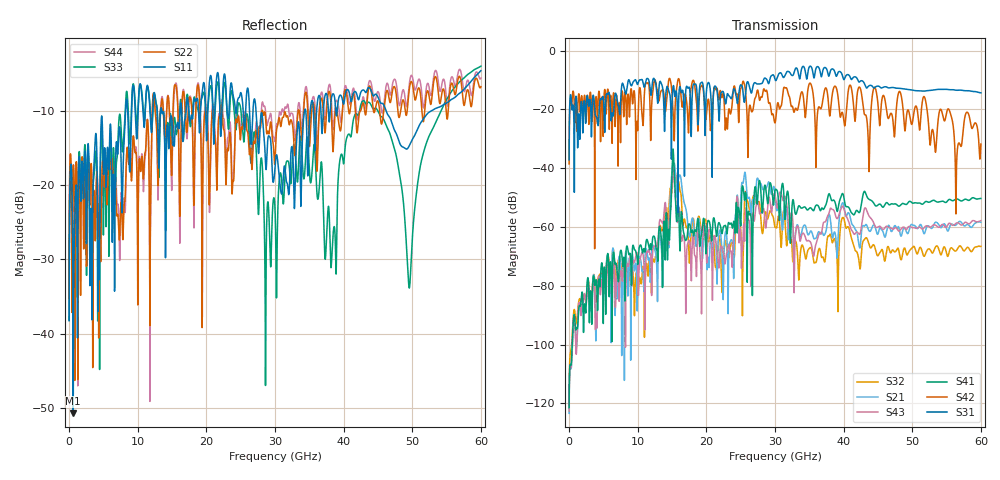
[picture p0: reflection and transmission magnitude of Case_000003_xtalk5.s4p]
! Info: Touchstone file created by circ.  Input file=CasetestDOE_NRZ_template_000003.circ
# Hz S RI R 50
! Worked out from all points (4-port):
!   6000 points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, 10 MHz to 60 GHz, reference 50 ohm
!   strongest paths, dB at 10 MHz, 15.01 GHz, 30.01 GHz, 45.01 GHz, 60 GHz:
!     S31: -37.1, -18.3, -9.8, -12.1, -14.4
!     S42: -38.6, -14.8, -24.6, -18.3, -31.8
!     S41: -121.4, -40.7, -47.5, -52.5, -50.3
!     S43: -122.6, -43.5, -49.2, -60.0, -57.9
!     S21: -123.4, -40.4, -48.7, -62.3, -58.4
!     S32: -120.6, -46.8, -60.1, -69.8, -66.6
!   lowest |S11| = -50.7 dB at 610 MHz (marker M1), VSWR 1.01, Z = 50.3 - j0.0177 ohm
!   |S11| at or under -10 dB: start of sweep to 8.241 GHz; 27.24 GHz to 34.32 GHz (7.08 GHz wide, 23 % of centre); 46.18 GHz to 52.85 GHz (6.665 GHz wide, 13.5 % of centre)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
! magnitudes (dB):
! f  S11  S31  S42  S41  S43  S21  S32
! 10 MHz  -38.3  -37.1  -38.6  -121.4  -122.6  -123.4  -120.6
! 610 MHz  -50.7  -18.8  -13.8  -92.4  -93.6  -93.7  -90.8
! 12.74 GHz  -9.3  -13.3  -12.3  -67.6  -67.0  -71.9  -70.6
! 15.23 GHz  -14.5  -12.0  -23.7  -36.0  -41.4  -39.2  -42.8
! 20.29 GHz  -8.4  -10.9  -16.5  -57.8  -62.2  -70.8  -64.6
! 49.56 GHz  -14.7  -13.3  -21.2  -51.3  -59.8  -60.9  -68.2
! 60 GHz  -4.6  -14.4  -31.8  -50.3  -57.9  -58.4  -66.6
